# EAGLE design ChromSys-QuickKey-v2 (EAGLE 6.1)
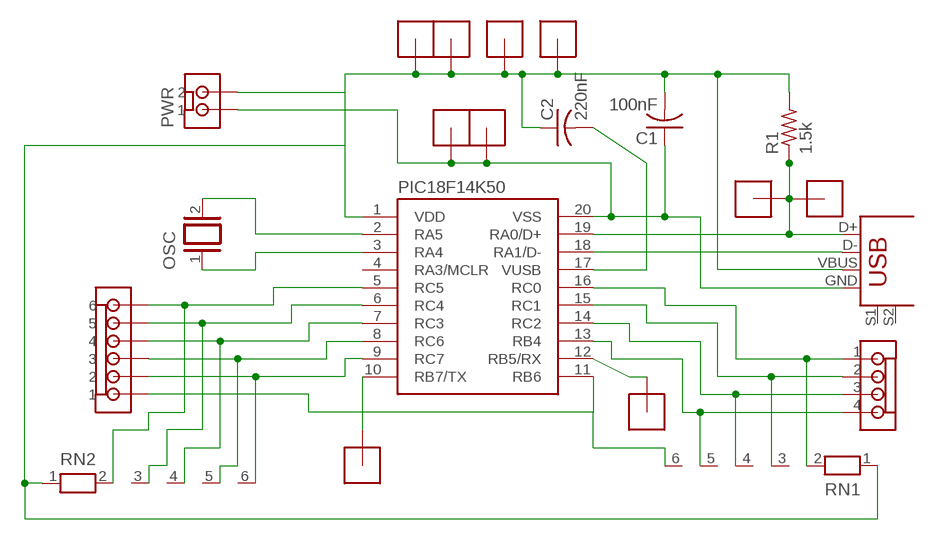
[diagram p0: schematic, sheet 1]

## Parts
C1  100nF  C-US050-024X044  [C050-024X044]
C2  220nF  C-US050-024X044  [C050-024X044]
G1  1HEADER  [J1]
G2  1HEADER  [J1]
HEADER1-4  KK4PIN  [KK4PIN]
HEADER5-10  MOLEXKK6  [MOLEXKK6]
J1  1HEADER  [J1]
J2  1HEADER  [J1]
OSC  XTAL/S  [QS]
P1  1HEADER  [J1]
P2  1HEADER  [J1]
P3  1HEADER  [J1]
P4  1HEADER  [J1]
PIC18F14K50  PIC18F14K50  [DIP-20]
PWR  MOLEXKK  [MOLEXKK]
R1  1.5k  R-US_0204/7  [0204/7]
RN1  RN05  [RN-6]
RN2  RN05  [RN-6]
RX  1HEADER  [J1]
TX  1HEADER  [J1]
USB  USB+SHIELD  [USB-B-PTH]

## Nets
N$1: OSC.2 PIC18F14K50.2(RA5)
N$2: OSC.1 PIC18F14K50.3(RA4)
N$3: J1.2(J1) J2.2(J1) PIC18F14K50.19(RA0/D+) R1.1 USB.D+
N$4: PIC18F14K50.18(RA1/D-) USB.D-
N$5: C1.2 C2.1 P1.2(J1) P2.2(J1) P3.2(J1) P4.2(J1) PIC18F14K50.1(VDD) PWR.1 R1.2 RN1.1 RN2.1 USB.VBUS
N$6: C1.1 G1.2(J1) G2.2(J1) PIC18F14K50.20(VSS) PWR.2 USB.GND
N$7: C2.2 PIC18F14K50.17(VUSB)
N$9: HEADER5-10.5 PIC18F14K50.6(RC4) RN2.3
N$10: HEADER5-10.4 PIC18F14K50.7(RC3) RN2.4
N$11: HEADER5-10.3 PIC18F14K50.8(RC6) RN2.5
N$12: HEADER5-10.2 PIC18F14K50.9(RC7) RN2.6
N$13: HEADER5-10.1 PIC18F14K50.11(RB6) RN1.6
N$14: HEADER1-4.1 PIC18F14K50.16(RC0) RN1.2
N$15: HEADER1-4.2 PIC18F14K50.15(RC1) RN1.3
N$16: HEADER1-4.3 PIC18F14K50.14(RC2) RN1.4
N$17: HEADER1-4.4 PIC18F14K50.13(RB4) RN1.5
N$18: PIC18F14K50.12(RB5/RX) RX.2(J1)
N$19: PIC18F14K50.10(RB7/TX) TX.2(J1)
N$21: HEADER5-10.6 PIC18F14K50.5(RC5) RN2.2
Unconnected: PIC18F14K50.4(RA3/MCLR) USB.S1 USB.S2

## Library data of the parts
C1 C2 = rcl:C-US: CAPACITOR, American symbol
G1 G2 J1 J2 P1-P4 RX TX = myFirst:1HEADER
HEADER1-4 = myFirst:KK4PIN
HEADER5-10 = myFirst:MOLEXKK6
OSC = special:XTAL/S: CRYSTAL
PIC18F14K50 = myFirst:PIC18F14K50
PWR = myFirst:MOLEXKK
R1 = rcl:R-US_: RESISTOR, American symbol
RN1 RN2 = resistor-net:RN05: RESISTOR NETWORK
USB = SparkFun:USB+SHIELD: USB+Shield USB connector with shield pins connectable

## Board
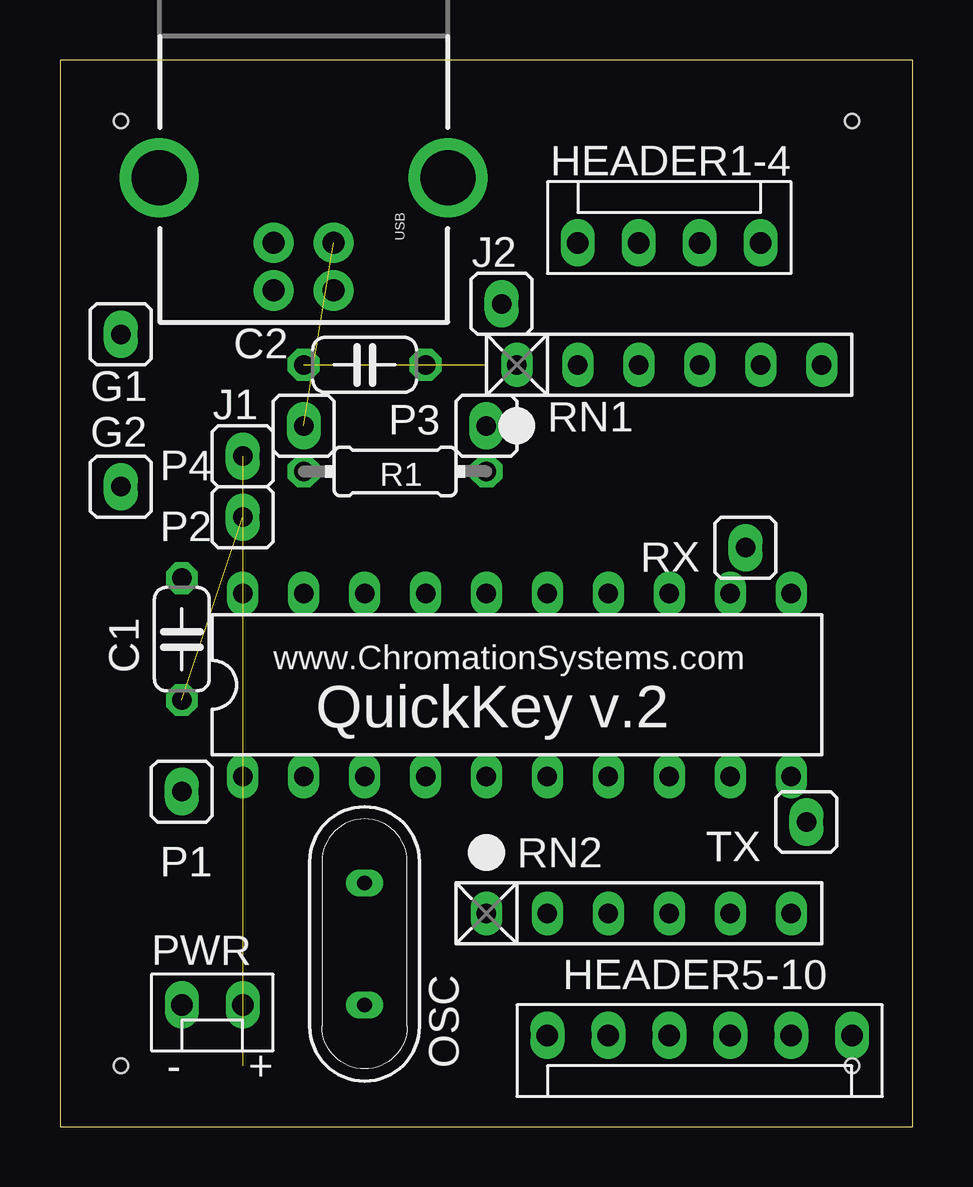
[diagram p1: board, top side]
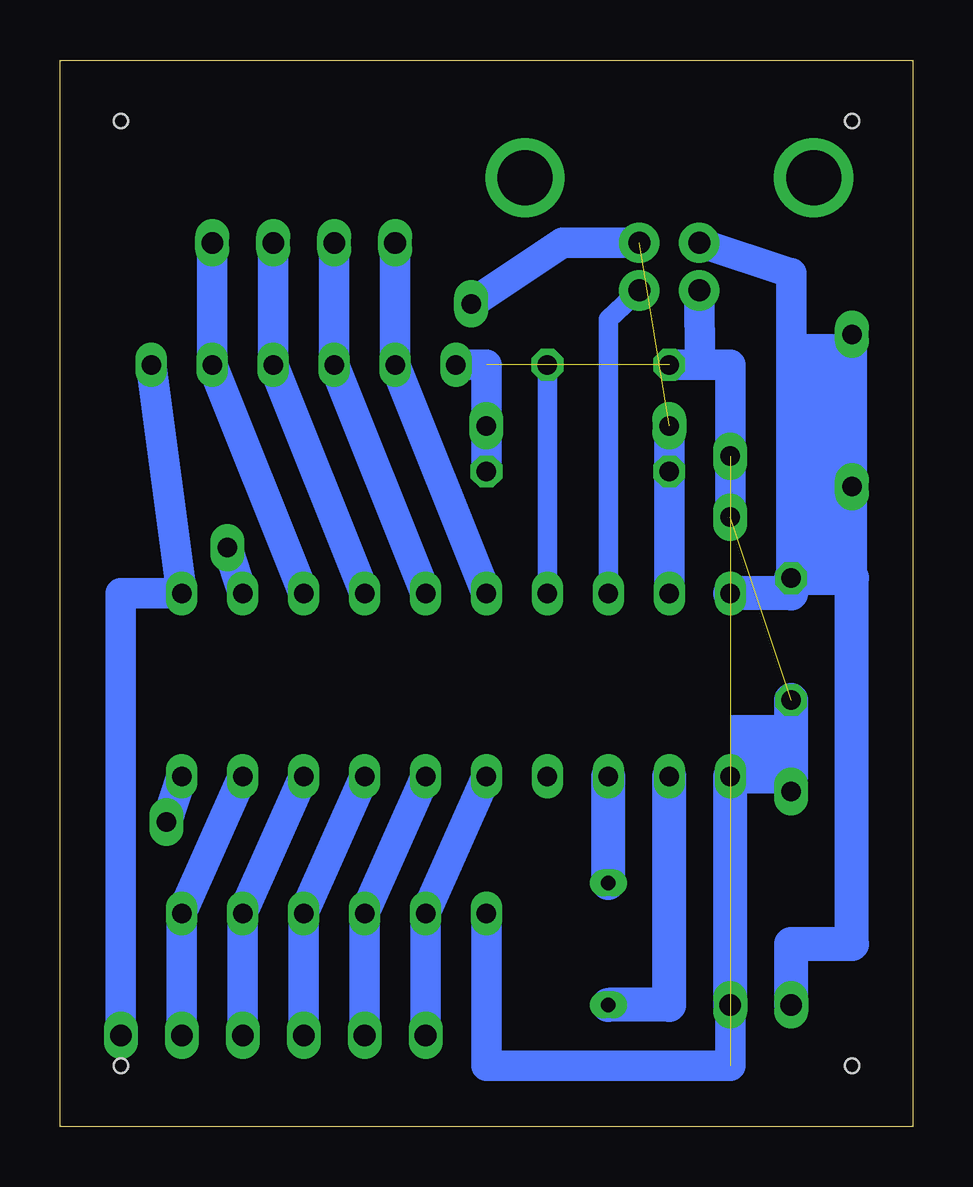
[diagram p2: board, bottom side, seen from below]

Size 35.56 x 44.45 mm. Coordinates in mm from the lower left corner, seen from the top.
Outline: 0,0 35.56,0 35.56,44.45 0,44.45 0,0
Copper layers (1*16): Top 0.035mm / dielectric 1.5mm / Bottom 0.035mm
Design rules: minimum track width 10mil, minimum drill 24mil, track to track 8mil, track to pad 8mil, pad to pad 8mil, via to via 8mil, smd to smd 8mil, copper to edge 40mil, drill to drill 6mil, minimum pad ring 10mil, minimum via ring 8mil, stop-mask expansion 4mil, vias tented up to drill 0mil, thermal gap 10mil
Holes 0.6 mm at 2.54,2.54 2.54,41.91 33.02,41.91 33.02,2.54

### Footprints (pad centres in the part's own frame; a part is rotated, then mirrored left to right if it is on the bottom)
C050-024X044 = drill 0.813 octagon: 1 -2.54,0; 2 2.54,0
J1 = drill 0.813 pad 1.422 long: 2 0,0
KK4PIN = drill 0.9 long: 1 -3.81,0; 2 -1.27,0; 3 1.27,0; 4 3.81,0
MOLEXKK6 = drill 0.9 long: 1 -6.35,0; 2 -3.81,0; 3 -1.27,0; 4 1.27,0; 5 3.81,0; 6 6.35,0
QS = drill 0.61 long: 1 -2.54,0; 2 2.54,0
DIP-20 = drill 0.813 long: 1 -11.43,-3.81; 2 -8.89,-3.81; 3 -6.35,-3.81; 4 -3.81,-3.81; 5 -1.27,-3.81; 6 1.27,-3.81; 7 3.81,-3.81; 8 6.35,-3.81; 9 8.89,-3.81; 10 11.43,-3.81; 11 11.43,3.81; 12 8.89,3.81; 13 6.35,3.81; 14 3.81,3.81; 15 1.27,3.81; 16 -1.27,3.81; 17 -3.81,3.81; 18 -6.35,3.81; 19 -8.89,3.81; 20 -11.43,3.81
MOLEXKK = drill 0.9 long: 1 -1.27,0; 2 1.27,0
0204/7 = drill 0.813 octagon: 1 -3.81,0; 2 3.81,0
RN-6 = drill 0.813 long: 1 -6.35,0; 2 -3.81,0; 3 -1.27,0; 4 1.27,0; 5 3.81,0; 6 6.35,0
USB-B-PTH = drill 0.914 pad 1.676: D+ 0,1.25; D- 1.981,1.25; GND 0,-1.25; VBUS 1.981,-1.25 | drill 2.286: S1 -2.718,-6.02; S2 -2.718,6.02

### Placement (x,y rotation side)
C1  5.08,20.32 270 top
C2  12.7,31.75 0 top
G1  2.54,33.02 90 top
G2  2.54,26.67 90 top
HEADER1-4  25.4,36.83 0 top
HEADER5-10  26.67,3.81 180 top
J1  10.16,29.21 270 top
J2  18.41,34.29 90 top
OSC  12.7,7.62 270 top
P1  5.08,13.97 90 top
P2  7.62,25.4 90 top
P3  17.78,29.21 90 top
P4  7.62,27.94 90 top
PIC18F14K50  19.05,18.41 0 top
PWR  6.35,5.08 180 top
R1  13.97,27.3 0 top
RN1  25.4,31.75 0 top
RN2  24.13,8.89 0 top
RX  28.57,24.13 90 top
TX  31.11,12.7 90 top
USB  10.16,36.83 270 top

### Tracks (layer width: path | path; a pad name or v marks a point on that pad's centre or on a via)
N$1
  Bottom 1.422: OSC.2 10.16,5.08 PIC18F14K50.2
N$2
  Bottom 1.422: OSC.1 PIC18F14K50.3
N$3  (1 unrouted)
  Bottom 1.27: PIC18F14K50.19 R1.1 J1.2 | USB.D+ 14.61,36.83 J2.2
N$4
  Bottom 0.813: PIC18F14K50.18 12.7,33.66 USB.D-
N$5  (3 unrouted)
  Bottom 0.813: C2.1 8.89,31.75
  Bottom 1.27: RN2.1 17.78,2.54 7.62,2.54 PWR.1 | 8.89,31.75 USB.VBUS | 5.08,14.61 P1.2 | P2.2 7.62,31.75 C2.1 | RN1.1 17.78,31.75 R1.2 P3.2
  Bottom 1.422: C1.2 5.08,14.61 PIC18F14K50.1 PWR.1
N$6
  Bottom 1.27: USB.GND 5.08,35.56 5.08,22.23 G2.2 | 2.54,22.86 G2.2 | G2.2 G1.2
  Bottom 1.422: PIC18F14K50.20 5.08,22.23 C1.1 2.54,22.86 2.54,7.62 5.08,7.62 PWR.2
N$7
  Bottom 0.813: PIC18F14K50.17 C2.2
N$9
  Bottom 1.27: PIC18F14K50.6 RN2.3 HEADER5-10.5
N$10
  Bottom 1.27: HEADER5-10.4 RN2.4 PIC18F14K50.7
N$11
  Bottom 1.27: PIC18F14K50.8 RN2.5 HEADER5-10.3
N$12
  Bottom 1.27: PIC18F14K50.9 RN2.6 HEADER5-10.2
N$13
  Bottom 1.27: RN1.6 PIC18F14K50.11 33.02,22.23 HEADER5-10.1
N$14
  Bottom 1.27: PIC18F14K50.16 RN1.2 HEADER1-4.1
N$15
  Bottom 1.27: PIC18F14K50.15 RN1.3 HEADER1-4.2
N$16
  Bottom 1.27: PIC18F14K50.14 RN1.4 HEADER1-4.3
N$17
  Bottom 1.27: HEADER1-4.4 RN1.5 PIC18F14K50.13
N$18
  Bottom 1.27: PIC18F14K50.12 RX.2
N$19
  Bottom 1.27: TX.2 PIC18F14K50.10
N$21
  Bottom 1.27: HEADER5-10.6 RN2.2 PIC18F14K50.5
(copper drawn outside any net)
  shapes: Bottom area x2

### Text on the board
tNames: www.ChromationSystems.com | QuickKey v.2 | HEADER5-10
